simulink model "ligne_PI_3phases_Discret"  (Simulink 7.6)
settings: Solver=ode3  StartTime=0.0  StopTime=0.02  RelTol=1e-3
InitFcn:
  | clc
  | close all
  | delete *.mat
StopFcn:
  | load Ia_Ua.mat
  | plotyy(x(1,:),x(2,:),x(1,:),x(3,:))
  | grid
  | title('Tension et courant - Phase A')
  | xlabel('temps')
libraries: powerlib x7

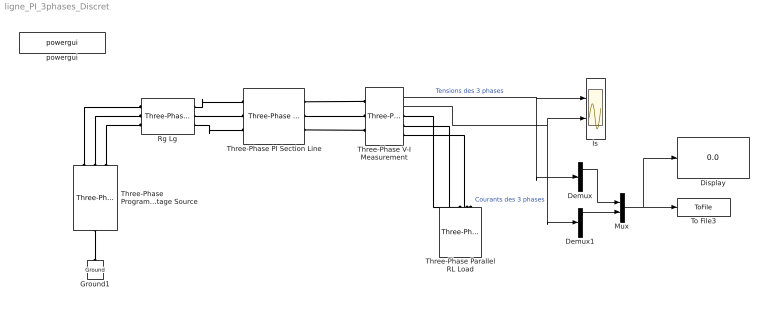
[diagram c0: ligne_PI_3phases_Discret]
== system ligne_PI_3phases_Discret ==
  Demux : Demux  Outputs=3
  Demux1 : Demux  Outputs=3
  Display : Display
  Ground1 : powerlib/Elements/Ground  DialogController=POWERSYS.PowerSysDialog  PhysicalDomain=powersysdomain  SubClassName=unknown  LeftPortType=p1  RightPortType=p1  LConnTagsString=a
  Is : Scope  NumInputPorts=2
  Mux : Mux  Inputs=2
  Rg Lg : powerlib/Elements/Three-Phase Parallel RLC Branch  DialogController=POWERSYS.PowerSysDialog  PhysicalDomain=powersysdomain  SubClassName=unknown  LeftPortType=p1  RightPortType=p1  LConnTagsString=A|B|C  RConnTagsString=A|B|C  BranchType=RL  Resistance=1  Inductance=1e-3  Capacitance=1e-6  Measurements=None
  Three-Phase PI Section Line : powerlib/Elements/Three-Phase PI Section Line  DialogController=POWERSYS.PowerSysDialog  PhysicalDomain=powersysdomain  SubClassName=unknown  LeftPortType=p1  RightPortType=p1  LConnTagsString=a|b|c  RConnTagsString=A|B|C  Frequency=60  Resistances=[ 0.01273 0.3864]  Inductances="[ 0.9337e-3  4.1264e-3]"  Capacitances=[12.74e-9 7.751e-9]  Length=150
  Three-Phase Parallel RL Load : powerlib/Elements/Three-Phase Parallel RLC Load  DialogController=POWERSYS.PowerSysDialog  PhysicalDomain=powersysdomain  SubClassName=unknown  LeftPortType=p1  RightPortType=p1  LConnTagsString=A|B|C  Configuration=Y (grounded)  NominalVoltage=230/sqrt(2)  NominalFrequency=60  ActivePower=1e3  InductivePower=10  CapacitivePower=0  Measurements=None
  Three-Phase Programmable Voltage Source : powerlib/Electrical Sources/Three-Phase Programmable Voltage Source  DialogController=POWERSYS.PowerSysDialog  SystemSampleTime=-1  PositiveSequence="[220e6/sqrt(2)  0 60]"  VariationEntity=None  VariationType=Step  VariationStep=0.5  VariationRate=10  VariationMagnitude=0.3  VariationFrequency=2  VariationTiming=[1 2]  VariationPhaseA=off  Amplitudes=[1 0.8 1.2 1.0]  TimeValues=[0 0.1 0.15 0.2]  HarmonicGeneration=off  HarmonicA=[3 0.2 -25 0]  HarmonicB=[2 0.15 35 2]  Timing="[0.05  3]"
  Three-Phase V-I Measurement : powerlib/Measurements/Three-Phase V-I Measurement  DialogController=POWERSYS.PowerSysDialog  SystemSampleTime=-1  VoltageMeasurement=phase-to-ground  SetLabelV=off  LabelV=Vabc  Vpu=off  VpuLL=off  CurrentMeasurement=yes  SetLabelI=off  LabelI=Iabc  Ipu=off  Pbase=100e6  Vbase=500e3  OutputType=Complex  PhasorSimulation=off  PSBequivalent=0
  To File3 : ToFile  Filename=Ia_Ua  MatrixName=x
  powergui : powerlib/powergui  Priority=1  SystemSampleTime=-1  SimulationMode=Discrete  SampleTime=50e-6  frequency=60  SPID=off  DisableSnubberDevices=off  DisableRonSwitches=off  DisableVfSwitches=off  SwTol=0  Interpol=off  frequencyindice=60  echomessages=off  HookPort=off  DisplayEquations=off  FunctionMessages=off  EnableUseOfTLC=off  x0status=blocks  RestoreLinks=warning  ResistiveCurrentMeasurement=off  Frange=[0:2:200]  Ylog=off  Xlog=on  ShowGrid=on  save=off  variable=ZData  structure=ScopeData  ZoomFFT=off  StartTime=0.0  cycles=1  DisplayStyle=1  fundamental=60  FreqAxis=off  MaxFrequency=1000  frequencyindicesteady=1  display=off  methode=off
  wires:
  Three-Phase V-I Measurement/1 -> Is/1, Demux/1  "Tensions des 3 phases"
  Three-Phase V-I Measurement/2 -> Is/2, Demux1/1  "Courants des 3 phases"
  Demux/1 -> Mux/1
  Demux1/1 -> Mux/2
  Mux/1 -> To File3/1, Display/1
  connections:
  Three-Phase Programmable Voltage Source/LConn1 -- Ground1/LConn1
  Three-Phase Programmable Voltage Source/RConn1 -- Rg Lg/LConn1
  Three-Phase Programmable Voltage Source/RConn2 -- Rg Lg/LConn2
  Three-Phase Programmable Voltage Source/RConn3 -- Rg Lg/LConn3
  Rg Lg/RConn1 -- Three-Phase PI Section Line/LConn1
  Rg Lg/RConn2 -- Three-Phase PI Section Line/LConn2
  Rg Lg/RConn3 -- Three-Phase PI Section Line/LConn3
  Three-Phase PI Section Line/RConn1 -- Three-Phase V-I Measurement/LConn1
  Three-Phase PI Section Line/RConn2 -- Three-Phase V-I Measurement/LConn2
  Three-Phase PI Section Line/RConn3 -- Three-Phase V-I Measurement/LConn3
  Three-Phase V-I Measurement/RConn3 -- Three-Phase Parallel RL Load/LConn3
  Three-Phase V-I Measurement/RConn2 -- Three-Phase Parallel RL Load/LConn2
  Three-Phase V-I Measurement/RConn1 -- Three-Phase Parallel RL Load/LConn1
